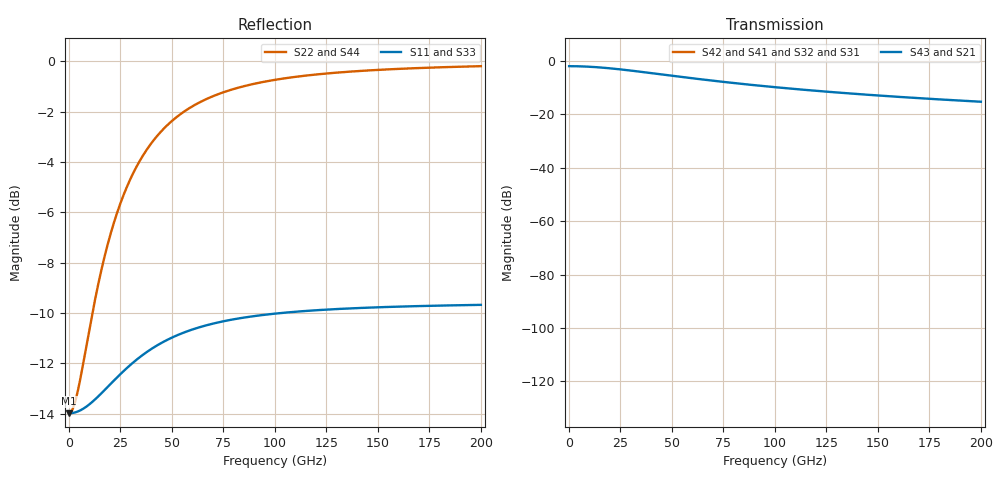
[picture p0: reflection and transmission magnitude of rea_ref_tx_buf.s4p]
! Created with skrf 1.10.0 (http://scikit-rf.org).
# Hz S RI R 50.0
!freq ReS11 ImS11 ReS12 ImS12 ReS13 ImS13
! ReS14 ImS14
! ReS21 ImS21 ReS22 ImS22 ReS23 ImS23
! ReS24 ImS24
! ReS31 ImS31 ReS32 ImS32 ReS33 ImS33
! ReS34 ImS34
! ReS41 ImS41 ReS42 ImS42 ReS43 ImS43
! ReS44 ImS44
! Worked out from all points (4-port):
!   2000 points, 100 MHz to 200 GHz, reference 50 ohm
!   strongest paths, dB at 100 MHz, 50.1 GHz, 100.1 GHz, 150.1 GHz, 200 GHz:
!     S43: -1.9, -5.5, -9.8, -12.9, -15.3
!     S21: -1.9, -5.5, -9.8, -12.9, -15.3
!     S42: -, -, -, -, -
!     S41: -, -, -, -, -
!     S32: -, -, -, -, -
!     S31: -, -, -, -, -
!   lowest |S11| = -14.0 dB at 100 MHz (marker M1), VSWR 1.50, Z = 75 - j0.188 ohm
!   |S11| at or under -10 dB: start of sweep to 102.7 GHz
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1e8  0.2 -0.00121  0.8 -0.00181  0 0  0 0
     0.8 -0.00181  0.2 -0.00271  0 0  0 0
     0 0  0 0  0.2 -0.00121  0.8 -0.00181
     0 0  0 0  0.8 -0.00181  0.2 -0.00271
9.2e9  0.1779 -0.1064  0.7668 -0.1596  0 0  0 0
       0.7668 -0.1596  0.1502 -0.2394  0 0  0 0
       0 0  0 0  0.1779 -0.1064  0.7668 -0.1596
       0 0  0 0  0.7668 -0.1596  0.1502 -0.2394
2.04e10  0.1064 -0.2029  0.6596 -0.3043  0 0  0 0
         0.6596 -0.3043  -0.0107 -0.4565  0 0  0 0
         0 0  0 0  0.1064 -0.2029  0.6596 -0.3043
         0 0  0 0  0.6596 -0.3043  -0.0107 -0.4565
4.07e10  -0.0447 -0.2658  0.433 -0.3986  0 0  0 0
         0.433 -0.3986  -0.3505 -0.598  0 0  0 0
         0 0  0 0  -0.0447 -0.2658  0.433 -0.3986
         0 0  0 0  0.433 -0.3986  -0.3505 -0.598
6.47e10  -0.1636 -0.2484  0.2546 -0.3727  0 0  0 0
         0.2546 -0.3727  -0.618 -0.559  0 0  0 0
         0 0  0 0  -0.1636 -0.2484  0.2546 -0.3727
         0 0  0 0  0.2546 -0.3727  -0.618 -0.559
9.47e10  -0.2379 -0.2044  0.1432 -0.3066  0 0  0 0
         0.1432 -0.3066  -0.7853 -0.46  0 0  0 0
         0 0  0 0  -0.2379 -0.2044  0.1432 -0.3066
         0 0  0 0  0.1432 -0.3066  -0.7853 -0.46
2e11  -0.3085 -0.1124  0.0373 -0.1686  0 0  0 0
      0.0373 -0.1686  -0.9441 -0.2529  0 0  0 0
      0 0  0 0  -0.3085 -0.1124  0.0373 -0.1686
      0 0  0 0  0.0373 -0.1686  -0.9441 -0.2529
